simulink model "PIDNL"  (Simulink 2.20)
settings: Solver=VariableStepDiscrete  StartTime=0.0  StopTime=10.0  RelTol=1e-3  AbsTol=1e-6
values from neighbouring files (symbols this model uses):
  a = input('Inserisci il dato da graficare [1=PIDNL 2=PD 3=PID]: ')    [grp.m]    (also in grp1.m = input('Inserisci il dato da graficare [1..3]'))
undefined symbols (not defined in the file or in its folder): b, NL
libraries: Puma x2

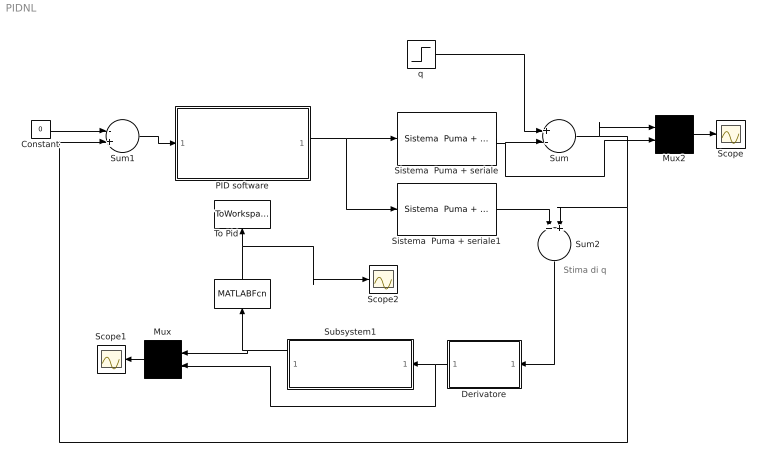
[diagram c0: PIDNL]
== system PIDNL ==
  note: Stima di q
  " " : MATLABFcn  Orientation=up  MATLABFcn=NL(u)  OutputWidth=-1
  Constant : Constant  Value=0
  Derivatore : Subsystem  Orientation=left  mask(Simulazione Derivatore implementato in maniera software){Td=0.13, T=0.030, N=5}
      mask prompts: Td "Costante di derivazione Td"; T "Sample Time T del PD"; N "Indice polo del derivatore [5..10]"
      mask init:
      | Kbeta=Td/(N*T+Td);
      | Kalfa=N*Kbeta;
  Mux : Mux  Orientation=left  Inputs=2
  Mux2 : Mux  Inputs=2
  PID software : Subsystem  mask(PID simulazione di una implementazione software.){Ti=a(size(a,1)), Td=0.17, T=.07, Kp=0.4, N=10}
      mask prompts: Ti "Costante integrativa Ti"; Td "Costante derivativa Td"; T "Sample Time del PID"; Kp "Costante proporzionale Kp"; N "Indice polo del derivatore [5..10]"
      mask init:
      | Kalfa=T/Ti;
      | Kgamma=Td/(N*T+Td);		Kbeta=N*Kgamma;
      | 
      | q0=Kp*(1+Kbeta);
      | q1=-Kp*(1+Kgamma-Kalfa+2*Kbeta);
      | q2=Kp*(Kgamma-Kalfa*Kgamma+Kbeta);
      | 
      | r1=Kgamma+1;
      | r2=Kgamma;
  Scope : Scope
  Scope1 : Scope
  Scope2 : Scope
  Sistema  Puma + seriale : Puma/Sistema  Puma + seriale  Ts=.260
  Sistema  Puma + seriale1 : Puma/Sistema  Puma + seriale  Ts=.260
  Subsystem1 : Subsystem  Orientation=left  mask(Filtro di Butterworth){ordine=5, freq=0.5/16}
      mask prompts: ordine "Ordine del filtro"; freq "Parametro K per ricavare la Freq. di taglio Ft"
      mask help: Attenzione! Considerare il parametro Fc come la frequanza di campionamento del segnale di ingresso, per cui la frequanza di taglio diviene Ft=K*Fc;
      mask init:
      | [b,a]=butter(ordine,freq);
  Sum : Sum  Inputs=+-
  Sum1 : Sum  Inputs=-+
  Sum2 : Sum  Orientation=down  Inputs=++
  To Pid : ToWorkspace  VariableName=Ti  SampleTime=-1
  q : Step  Time=.1  Before=0  After=45
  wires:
  PID software/1(Out1) -> Sistema  Puma + seriale/1, Sistema  Puma + seriale1/1
  Constant/1 -> Sum1/1
  q/1 -> Sum/1
  Sistema  Puma + seriale1/1 -> Sum2/1
  Mux2/1 -> Scope/1
  Sum/1 -> Sum1/2, Sum2/2, Mux2/1
  Sistema  Puma + seriale/1 -> Sum/2, Mux2/2
  Sum1/1 -> PID software/1(In1)
  Sum2/1 -> Derivatore/1(In1)
  Mux/1 -> Scope1/1
  Derivatore/1(Out1) -> Subsystem1/1(In1), Mux/2
  Subsystem1/1(Out1) -> Mux/1, " "/1
  " "/1 -> To Pid/1, Scope2/1

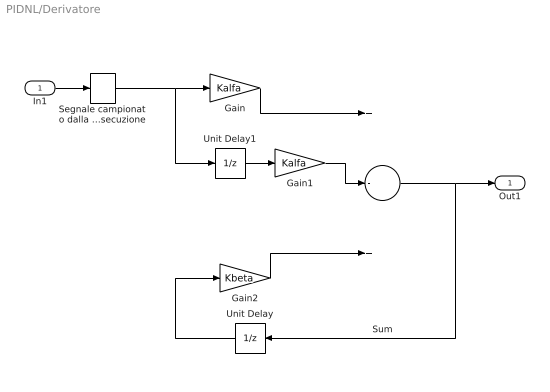
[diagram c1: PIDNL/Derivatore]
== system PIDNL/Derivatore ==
  In1 : Inport  Port=1  PortWidth=-1  SampleTime=-1
  Gain : Gain  Gain=Kalfa
  Gain1 : Gain  Gain=Kalfa
  Gain2 : Gain  Gain=Kbeta
  Segnale campionato dalla procedura software al momento ciclo  di'esecuzione : ZeroOrderHold  SampleTime=T
  Sum : Sum  Inputs=+-+
  Unit Delay : UnitDelay  Orientation=left  X0=0  SampleTime=T
  Unit Delay1 : UnitDelay  X0=0  SampleTime=T
  Out1 : Outport  Port=1
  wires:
  Gain1/1 -> Sum/2
  Unit Delay/1 -> Gain2/1
  Gain2/1 -> Sum/3
  Gain/1 -> Sum/1
  Unit Delay1/1 -> Gain1/1
  Sum/1 -> Out1/1, Unit Delay/1
  In1/1 -> Segnale campionato dalla procedura software al momento ciclo  di'esecuzione/1
  Segnale campionato dalla procedura software al momento ciclo  di'esecuzione/1 -> Gain/1, Unit Delay1/1

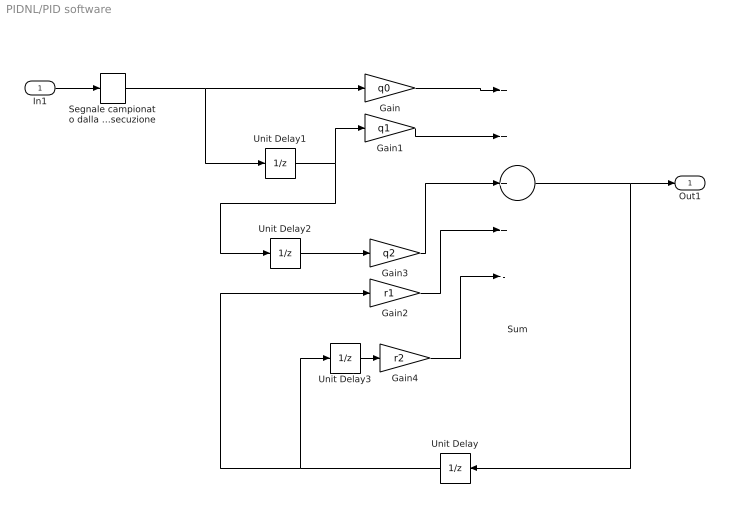
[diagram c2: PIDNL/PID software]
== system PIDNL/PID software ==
  In1 : Inport  Port=1  PortWidth=-1  SampleTime=-1
  Gain : Gain  Gain=q0
  Gain1 : Gain  Gain=q1
  Gain2 : Gain  Gain=r1
  Gain3 : Gain  Gain=q2
  Gain4 : Gain  Gain=r2
  Segnale campionato dalla procedura software al momento del  ciclo di esecuzione : ZeroOrderHold  SampleTime=T
  Sum : Sum  Inputs=++++-
  Unit Delay : UnitDelay  Orientation=left  X0=0  SampleTime=T
  Unit Delay1 : UnitDelay  X0=0  SampleTime=T
  Unit Delay2 : UnitDelay  X0=0  SampleTime=T
  Unit Delay3 : UnitDelay  X0=0  SampleTime=T
  Out1 : Outport  Port=1
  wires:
  Segnale campionato dalla procedura software al momento del  ciclo di esecuzione/1 -> Unit Delay1/1, Gain/1
  Gain4/1 -> Sum/5
  Unit Delay3/1 -> Gain4/1
  Unit Delay/1 -> Unit Delay3/1, Gain2/1
  Gain2/1 -> Sum/4
  Gain3/1 -> Sum/3
  Unit Delay2/1 -> Gain3/1
  Unit Delay1/1 -> Unit Delay2/1, Gain1/1
  Sum/1 -> Out1/1, Unit Delay/1
  Gain/1 -> Sum/1
  Gain1/1 -> Sum/2
  In1/1 -> Segnale campionato dalla procedura software al momento del  ciclo di esecuzione/1

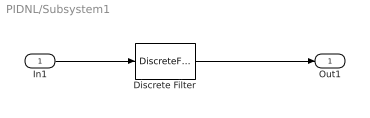
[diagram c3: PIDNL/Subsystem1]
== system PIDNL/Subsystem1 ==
  In1 : Inport  Port=1  PortWidth=-1  SampleTime=-1
  Discrete Filter : DiscreteFilter  Numerator=b  Denominator=a  SampleTime=.032
  Out1 : Outport  Port=1
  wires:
  In1/1 -> Discrete Filter/1
  Discrete Filter/1 -> Out1/1
